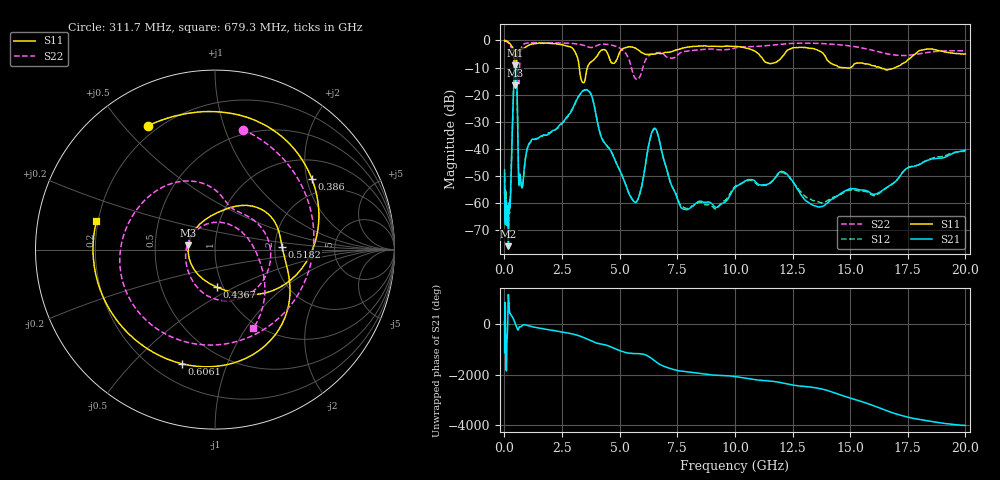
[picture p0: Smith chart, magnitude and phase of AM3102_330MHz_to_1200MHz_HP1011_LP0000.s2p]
! Date/Time: Tue, Sep 11, 2018 5:19 PM
! Network Analyzer: Agilent Technologies E8362B Rev: A.07.50.63
! Sweep from 0.010 to 20.000 GHz, 1601 Points, Sweep Type: LOG
! Power Supply: 4.949 V, 0.001 A
# Hz S DB R 50
!freq MagS11 AngS11 MagS21 AngS21 MagS12 AngS12 MagS22 AngS22
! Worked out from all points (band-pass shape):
!   1601 points, 10 MHz to 20 GHz, reference 50 ohm
!   highest |S21| = -9.19 dB at 478 MHz (marker M1); lowest = -75.9 dB at 172.1 MHz (marker M2)
!   |S21| within 3 dB of the highest: 428.9 MHz to 527.6 MHz (98.67 MHz wide, 20.6 % of centre)
!   lowest |S11| = -16.5 dB at 453.6 MHz (marker M3), VSWR 1.35, Z = 37.1 + j1.78 ohm
!   |S11| at or under -10 dB: 3.25 GHz to 3.599 GHz (349.5 MHz wide, 10.2 % of centre); 14.66 GHz to 15.02 GHz (362 MHz wide, 2.44 % of centre); 16.3 GHz to 16.96 GHz (656.4 MHz wide, 3.95 % of centre)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
!   |S22| runs from -16.5 to -0.1 dB; largest |S21 - S12| = 0.005
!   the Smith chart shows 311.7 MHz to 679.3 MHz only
!   S11 on the Smith chart (normalised r, x): 311.7 MHz: 0.16, +0.59; 386 MHz: 1.52, +2.15; 436.7 MHz: 0.94, -0.41; 518.2 MHz: 2.19, +0.08; 606.1 MHz: 0.31, -0.70; 679.3 MHz: 0.19, +0.11
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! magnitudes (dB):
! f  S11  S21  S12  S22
! 10 MHz  0.0  -49.0  -47.4  -0.1
! 35.55 MHz  0.0  -65.5  -63.2  -0.2
! 48.41 MHz  0.0  -57.2  -57.2  -0.3
! 126.4 MHz  -0.4  -67.7  -66.4  -0.6
! 172.1 MHz  -0.6  -75.9  -68.6  -0.9
! 311.7 MHz  -2.1  -43.7  -43.5  -3.3
! 386 MHz  -3.5  -21.3  -21.3  -5.5
! 436.7 MHz  -13.5  -11.2  -11.2  -5.6
! 447.2 MHz  -16.2  -10.1  -10.2  -5.9
! 453.6 MHz  -16.5  -9.7  -9.8  -6.1
! 478 MHz  -10.9  -9.2  -9.3  -7.1
! 518.2 MHz  -8.5  -10.8  -10.8  -11.7
! 606.1 MHz  -3.6  -47.1  -47.5  -14.5
! 679.3 MHz  -3.4  -49.6  -49.7  -6.2
! 1.59 GHz  -1.0  -35.3  -35.3  -0.8
! 3.617 GHz  -9.6  -18.5  -18.2  -2.3
! 5.652 GHz  -2.7  -59.6  -59.7  -13.7
! 6.487 GHz  -5.1  -32.5  -32.8  -4.8
! 7.882 GHz  -2.6  -62.4  -61.9  -4.0
! 12.03 GHz  -6.2  -48.3  -48.7  -1.4
! 13.74 GHz  -4.2  -61.3  -59.9  -1.1
! 20 GHz  -5.0  -40.4  -40.9  -3.8
